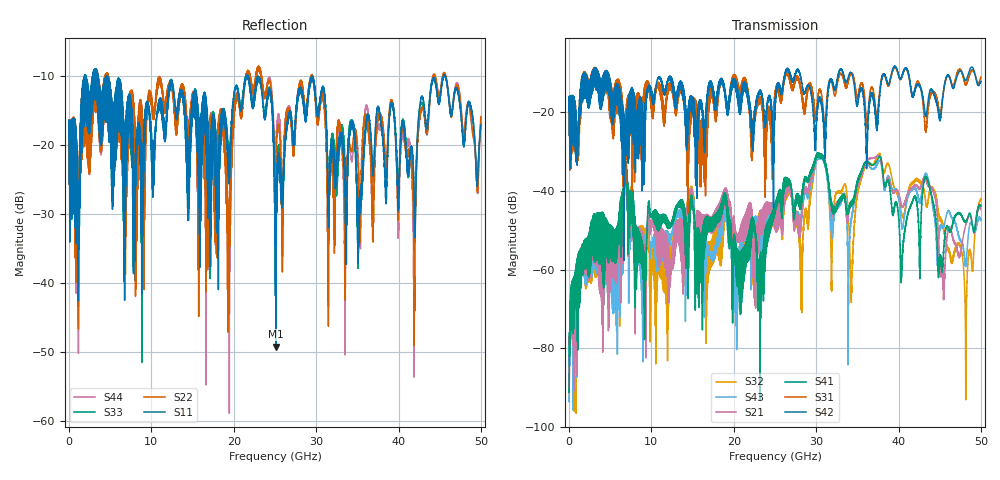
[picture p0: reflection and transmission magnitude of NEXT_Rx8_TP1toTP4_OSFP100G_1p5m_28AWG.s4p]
! Touchstone data
! Created: 27-Feb-2019 by IdEM 12 (12.1.0)
! COMMENTS
!  Created Wed Feb 27 09:43:39 2019
!  64 Port Network Data from SP1.SP block
!  freq  magS1_1  angS1_1  magS1_2  angS1_2  magS1_3  angS1_3  magS1_4  angS1_4
!  magS1_5  angS1_5  magS1_6  angS1_6  magS1_7  angS1_7  magS1_8  angS1_8
!  magS1_9  angS1_9  magS1_10  angS1_10  magS1_11  angS1_11  magS1_12  angS1_12
!  magS1_13  angS1_13  magS1_14  angS1_14  magS1_15  angS1_15  magS1_16  angS1_16
!  magS1_17  angS1_17  magS1_18  angS1_18  magS1_19  angS1_19  magS1_20  angS1_20
!  magS1_21  angS1_21  magS1_22  angS1_22  magS1_23  angS1_23  magS1_24  angS1_24
!  magS1_25  angS1_25  magS1_26  angS1_26  magS1_27  angS1_27  magS1_28  angS1_28
!  magS1_29  angS1_29  magS1_30  angS1_30  magS1_31  angS1_31  magS1_32  angS1_32
!  magS1_33  angS1_33  magS1_34  angS1_34  magS1_35  angS1_35  magS1_36  angS1_36
!  magS1_37  angS1_37  magS1_38  angS1_38  magS1_39  angS1_39  magS1_40  angS1_40
!  magS1_41  angS1_41  magS1_42  angS1_42  magS1_43  angS1_43  magS1_44  angS1_44
!  magS1_45  angS1_45  magS1_46  angS1_46  magS1_47  angS1_47  magS1_48  angS1_48
!  magS1_49  angS1_49  magS1_50  angS1_50  magS1_51  angS1_51  magS1_52  angS1_52
!  magS1_53  angS1_53  magS1_54  angS1_54  magS1_55  angS1_55  magS1_56  angS1_56
!  magS1_57  angS1_57  magS1_58  angS1_58  magS1_59  angS1_59  magS1_60  angS1_60
!  magS1_61  angS1_61  magS1_62  angS1_62  magS1_63  angS1_63  magS1_64  angS1_64
!  magS2_1  angS2_1  magS2_2  angS2_2  magS2_3  angS2_3  magS2_4  angS2_4
!  magS2_5  angS2_5  magS2_6  angS2_6  magS2_7  angS2_7  magS2_8  angS2_8
!  magS2_9  angS2_9  magS2_10  angS2_10  magS2_11  angS2_11  magS2_12  angS2_12
!  magS2_13  angS2_13  magS2_14  angS2_14  magS2_15  angS2_15  magS2_16  angS2_16
!  magS2_17  angS2_17  magS2_18  angS2_18  magS2_19  angS2_19  magS2_20  angS2_20
!  magS2_21  angS2_21  magS2_22  angS2_22  magS2_23  angS2_23  magS2_24  angS2_24
!  magS2_25  angS2_25  magS2_26  angS2_26  magS2_27  angS2_27  magS2_28  angS2_28
!  magS2_29  angS2_29  magS2_30  angS2_30  magS2_31  angS2_31  magS2_32  angS2_32
!  magS2_33  angS2_33  magS2_34  angS2_34  magS2_35  angS2_35  magS2_36  angS2_36
!  magS2_37  angS2_37  magS2_38  angS2_38  magS2_39  angS2_39  magS2_40  angS2_40
!  magS2_41  angS2_41  magS2_42  angS2_42  magS2_43  angS2_43  magS2_44  angS2_44
!  magS2_45  angS2_45  magS2_46  angS2_46  magS2_47  angS2_47  magS2_48  angS2_48
!  magS2_49  angS2_49  magS2_50  angS2_50  magS2_51  angS2_51  magS2_52  angS2_52
!  magS2_53  angS2_53  magS2_54  angS2_54  magS2_55  angS2_55  magS2_56  angS2_56
!  magS2_57  angS2_57  magS2_58  angS2_58  magS2_59  angS2_59  magS2_60  angS2_60
!  magS2_61  angS2_61  magS2_62  angS2_62  magS2_63  angS2_63  magS2_64  angS2_64
!  magS3_1  angS3_1  magS3_2  angS3_2  magS3_3  angS3_3  magS3_4  angS3_4
!  magS3_5  angS3_5  magS3_6  angS3_6  magS3_7  angS3_7  magS3_8  angS3_8
!  magS3_9  angS3_9  magS3_10  angS3_10  magS3_11  angS3_11  magS3_12  angS3_12
!  magS3_13  angS3_13  magS3_14  angS3_14  magS3_15  angS3_15  magS3_16  angS3_16
!  magS3_17  angS3_17  magS3_18  angS3_18  magS3_19  angS3_19  magS3_20  angS3_20
!  magS3_21  angS3_21  magS3_22  angS3_22  magS3_23  angS3_23  magS3_24  angS3_24
!  magS3_25  angS3_25  magS3_26  angS3_26  magS3_27  angS3_27  magS3_28  angS3_28
!  magS3_29  angS3_29  magS3_30  angS3_30  magS3_31  angS3_31  magS3_32  angS3_32
!  magS3_33  angS3_33  magS3_34  angS3_34  magS3_35  angS3_35  magS3_36  angS3_36
!  magS3_37  angS3_37  magS3_38  angS3_38  magS3_39  angS3_39  magS3_40  angS3_40
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# Hz S MA R 50
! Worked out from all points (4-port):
!   5000 points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, 10 MHz to 50 GHz, reference 50 ohm
!   strongest paths, dB at 10 MHz, 12.51 GHz, 25.01 GHz, 37.51 GHz, 50 GHz:
!     S42: -19.6, -12.0, -18.5, -21.3, -12.1
!     S31: -19.6, -14.0, -15.9, -19.1, -11.0
!     S41: -90.4, -47.8, -44.8, -31.8, -43.7
!     S21: -91.6, -56.3, -49.6, -31.0, -44.8
!     S43: -92.5, -50.6, -44.4, -32.8, -47.5
!     S32: -92.3, -54.3, -49.5, -30.8, -41.9
!   lowest |S11| = -49.2 dB at 25.11 GHz (marker M1), VSWR 1.01, Z = 50.3 + j0.113 ohm
!   |S11| at or under -10 dB: 4.66 GHz to 21.51 GHz (16.85 GHz wide, 129 % of centre); 22.94 GHz to 45.47 GHz (22.53 GHz wide, 65.9 % of centre); 45.68 GHz to end of sweep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
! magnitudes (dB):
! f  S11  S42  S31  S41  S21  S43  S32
! 10 MHz  -19.2  -19.6  -19.6  -90.4  -91.6  -92.5  -92.3
! 6.83 GHz  -17.8  -30.5  -23.0  -32.9  -34.0  -34.5  -35.7
! 25.11 GHz  -49.2  -15.8  -14.8  -44.1  -50.4  -43.9  -50.0
! 34.29 GHz  -16.5  -10.1  -10.2  -43.7  -43.2  -46.9  -64.5
! 37.64 GHz  -15.1  -17.0  -16.0  -31.3  -31.1  -32.3  -30.5
! 48.14 GHz  -17.6  -11.9  -12.9  -47.8  -48.8  -58.6  -77.0
! 50 GHz  -17.1  -12.1  -11.0  -43.7  -44.8  -47.5  -41.9
